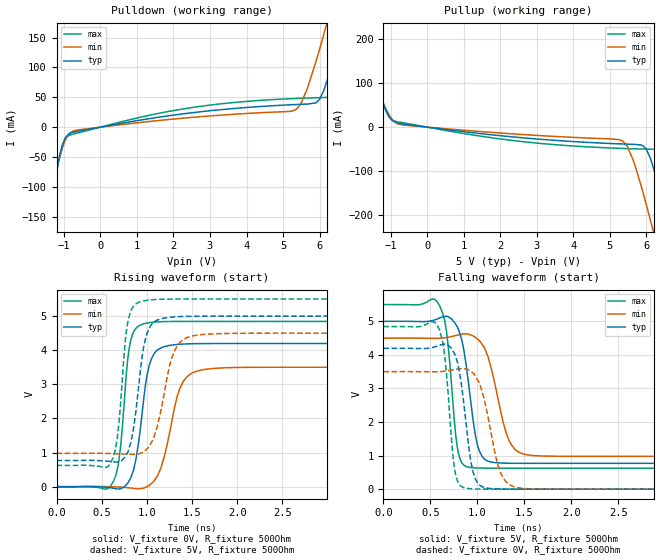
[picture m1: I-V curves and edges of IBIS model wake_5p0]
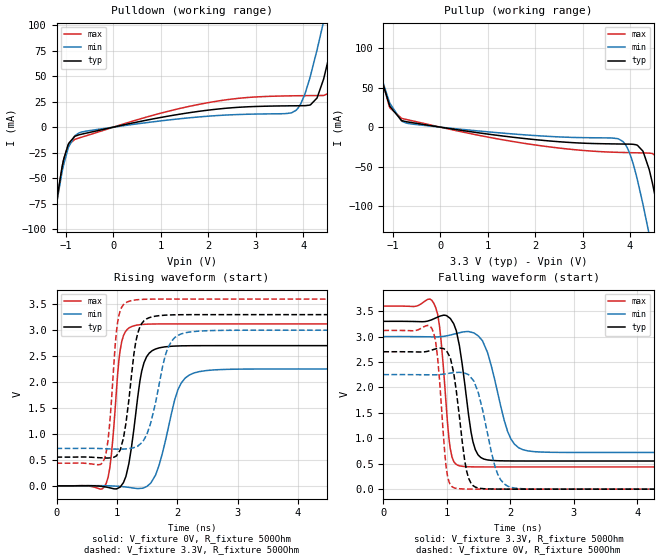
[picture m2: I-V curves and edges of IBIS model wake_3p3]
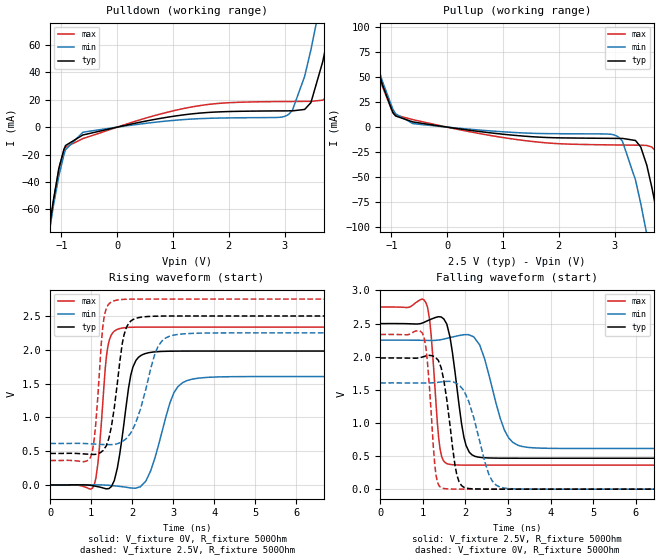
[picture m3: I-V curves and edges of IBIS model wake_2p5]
|Texas Instruments Incorporated
| Marketing part#   Digital Voltage Range   Package-type   #pins
|  TPL5110   1.8V - 5.0V   SOT23   6
[IBIS Ver]   4.1
[File name]   tpl5110.ibs
[File Rev]   1.0
[Date]   09/09/2014
[Source]
| Texas Instruments Incorporated.
| 12500 TI Blvd
| Dallas, TX -75243
[Notes]   Revision History:
| Rev 1.0: 09/09/2014
| - Initial version of the model
| - Model generated from simulations in TISPICE
| - C_comp although listed in numerical order of value are
|   obtained from varying PVT conditions. For PVT conditions for
|   each specific value refer the buffer description under
|   respective [Model]. IBIS model user is responsible for using
|   appropriate C_comp to simulate for Signal Integrity.
| - Warnings regarding combined Non-monotonicity of various models have been
|   reviewd and considered minor and can be ignored.
| - Model names with a trailing _1p8 contains the model for
|   1.8V operation.Model names with a trailing _2p5 contains the model for
|   2.5V operation.Model names with a trailing _3p3 contains the model for
|   3.3V operation.Model names with a trailing _5p0 contains the model
|   for 5.0V operation.
[Disclaimer]
| This model is designed as an aid for customers of Texas Instruments.
| TI and its licensors and suppliers make no warranties, either expressed
| or implied, with respect to this  model, including the warranties of
| merchantability or fitness for a particular purpose. The model is
| provided solely on an "as is" basis. The entire risk as to its quality
| and performance is with the customer.
[Copyright]
 (C) Copyright 2014 Texas Instruments Incorporated.All rights reserved.
|   Device
[Component] TPL5110
[Manufacturer]   TI
[Package]  |
|   typ   min   max
R_pkg   0.067   0.027   0.083
L_pkg   0.937nH   0.593nH   1.143nH
C_pkg   0.144pF   0.126pF   0.200pF
[Pin]  signal_name   model_name   R_pin   L_pin   C_pin
1   VDD   POWER   NA   NA   NA
2   GND   GND   NA   NA   NA
3   EN_oneshot done   NA   NA   NA
4   DONE   done   NA   NA   NA
5   WAKE_MDRV   wake   NA   NA   NA
6   MRST_DELAY   mrst   NA   NA   NA
|   Model Selectors
[Model Selector]  done
done_5p0  done buffer at 5.0V operation
done_3p3  done buffer at 3.3V operation
done_2p5  done buffer at 2.5V operation
done_1p8  done buffer at 1.8V operation
[Model Selector]  mrst
mrst_5p0  mrst buffer at 5.0V operation
mrst_3p3  mrst buffer at 3.3V operation
mrst_2p5  mrst buffer at 2.5V operation
mrst_1p8  mrst buffer at 1.8V operation
[Model Selector]  rstn
rstn_5p0  rstn buffer at 5.0V operation
rstn_3p3  rstn buffer at 3.3V operation
rstn_2p5  rstn buffer at 2.5V operation
rstn_1p8  rstn buffer at 1.8V operation
[Model Selector]  wake
wake_5p0  wake buffer at 5.0V operation
wake_3p3  wake buffer at 3.3V operation
wake_2p5  wake buffer at 2.5V operation
wake_1p8  wake buffer at 1.8V operation
| Models and submodels in the file (16): wake_5p0 (Output), wake_3p3 (Output), wake_2p5 (Output), wake_1p8 (Output), rstn_5p0 (I/O_open_drain), rstn_3p3 (I/O_open_drain), rstn_2p5 (I/O_open_drain), rstn_1p8 (I/O_open_drain), mrst_5p0 (Input), mrst_3p3 (Input), mrst_2p5 (Input), mrst_1p8 (Input), done_5p0 (I/O), done_3p3 (I/O), done_2p5 (I/O), done_1p8 (I/O)
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|   Model
[Model]   wake_5p0
Model_type   Output
Polarity   Non-Inverting
Vmeas = 2.5
Vref = 0
Cref = 1pF
Rref = 100000
|   typ   min   max
C_comp   0.327pF   0.289pF   0.359pF
[Voltage Range]   5   4.5   5.5
[Temperature Range]   25   105   -40
[Pullup Reference]   5   4.5   5.5
[Pulldown Reference]   0   0   0
[Power Clamp Reference]   5   4.5   5.5
[GND Clamp Reference]   0   0   0
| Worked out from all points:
|   slope of the pulldown table from 0 to 0.75 V, typ, clamps not added: 90.8 ohm
|   slope of the pullup table from 0 to 0.75 V, typ, clamps not added: 95.6 ohm
|   falling waveform, V_fixture 5V, R_fixture 500Ohm: 20-80 % time 124ps typ, 177ps min, 91.5ps max; typ from 5 V to 0.769 V
|   rising waveform, V_fixture 0V, R_fixture 500Ohm: 20-80 % time 129ps typ, 183ps min, 95.6ps max; typ from 0 V to 4.2 V
|   rising waveform, V_fixture 5V, R_fixture 500Ohm: 20-80 % time 123ps typ, 173ps min, 92.1ps max; typ from 0.769 V to 5 V
|   falling waveform, V_fixture 0V, R_fixture 500Ohm: 20-80 % time 113ps typ, 160ps min, 84.8ps max; typ from 4.2 V to 0 V
[Pulldown]
|   Voltage   I(typ)   I(min)   I(max)
-5V       -1.486A    -1.386A    -1.583A
-1.595V   -201.3mA   -192.2mA   -216.2mA
-1.43V    -144.2mA   -140.1mA   -154.1mA
-1.025V   -28.11mA   -32.78mA   -28.05mA
-710mV    -8.019mA   -5.887mA   -11.19mA
5.335V    37.79mA    29.02mA    47.98mA
5.905V    41.01mA    110.7mA    49.27mA
6.25V     86.31mA    185.2mA    49.89mA
6.595V    163.7mA    263.5mA    62.44mA
6.955V    251.3mA    347.1mA    139.6mA
7.33V     345.1mA    435.3mA    235.9mA
10V       1.032A     1.077A     962.9mA
[Pullup]
|   Voltage   I(typ)   I(min)   I(max)
-5V       1.028A     955.3mA    1.095A
-2.09V    266.5mA    250.1mA    284mA
-1.655V   156.9mA    149.7mA    165.6mA
-1.085V   30.71mA    34.2mA     29.01mA
-770mV    8.367mA    6.734mA    11.53mA
5.32V     -38.27mA   -30.34mA   -48.45mA
5.905V    -42.54mA   -148.5mA   -49.81mA
6.25V     -108.9mA   -257.7mA   -50.35mA
6.685V    -253.3mA   -403.2mA   -97.13mA
6.955V    -349.7mA   -495.6mA   -188.1mA
7.33V     -486.7mA   -625.3mA   -328.5mA
10V       -1.491A    -1.568A    -1.386A
[Ramp]
R_load = 500
|   typ   min   max
dV/dt_r   2.51801/1.28569e-10   2.10124/1.82749e-10   2.90712/9.55706e-11
dV/dt_f   2.53872/1.23628e-10   2.11358/1.77147e-10   2.92537/9.14795e-11
[Falling Waveform]
V_fixture = 5V
V_fixture_min = 4.5V
V_fixture_max = 5.5V
R_fixture = 500Ohm
C_fixture = 0F
|   Time   V(typ)   V(min)   V(max)
0s        5V         4.5V       5.5V
598ps     5.1V       4.497V     5.469V
672.4ps   5.148V     4.519V     4.695V
785.3ps   4.838V     4.589V     1.276V
913.9ps   2.991V     4.609V     651.2mV
984.6ps   1.53V      4.508V     633.3mV
1.05ns    978.3mV    4.319V     627.8mV
1.336ns   773.4mV    1.464V     624.5mV
1.532ns   769.5mV    1.022V     624.5mV
10ns      768.8mV    977.4mV    624.4mV
[Rising Waveform]
V_fixture = 0V
V_fixture_min = 0V
V_fixture_max = 0V
R_fixture = 500Ohm
C_fixture = 0F
|   Time   V(typ)   V(min)   V(max)
0s        11.88uV    -5.338uV   -17.74uV
632.2ps   -48.36mV   -3.24mV    167.3mV
691.1ps   -65.39mV   -11.2mV    773.4mV
818.4ps   245.1mV    -39.05mV   4.252V
906ps     1.246V     -61.22mV   4.702V
990.3ps   3.07V      -11.5mV    4.792V
1.154ns   4.065V     533.9mV    4.836V
1.403ns   4.182V     3.087V     4.845V
1.659ns   4.195V     3.445V     4.845V
10ns      4.197V     3.502V     4.845V
[Rising Waveform]
V_fixture = 5V
V_fixture_min = 4.5V
V_fixture_max = 5.5V
R_fixture = 500Ohm
C_fixture = 0F
|   Time   V(typ)   V(min)   V(max)
0s        768.8mV    977.4mV    624.4mV
598ps     740.3mV    971.7mV    683.4mV
672.4ps   723.3mV    964.8mV    1.418V
759.4ps   874.6mV    956.6mV    4.228V
800.1ps   1.102V     952.8mV    4.955V
990.3ps   4.391V     1.079V     5.46V
1.116ns   4.884V     1.766V     5.491V
1.308ns   4.978V     3.993V     5.499V
1.532ns   4.997V     4.432V     5.5V
10ns      5V         4.5V       5.5V
[Falling Waveform]
|Gnd
V_fixture = 0V
V_fixture_min = 0V
V_fixture_max = 0V
R_fixture = 500Ohm
C_fixture = 0F
|   Time   V(typ)   V(min)   V(max)
0s        4.197V     3.502V     4.845V
571.1ps   4.261V     3.498V     4.895V
652.5ps   4.32V      3.517V     3.999V
759.4ps   4.021V     3.564V     575.3mV
884.9ps   1.85V      3.576V     24.89mV
947.8ps   590.7mV    3.476V     8.984mV
1.002ns   194.8mV    3.261V     4.297mV
1.253ns   5.124mV    456.9mV    268.3uV
1.44ns    760.1uV    39.68mV    262.3uV
10ns      -8.208uV   6.088uV    -12.22uV
|   Model
[Model]   wake_3p3
Model_type   Output
Polarity   Non-Inverting
Vmeas = 1.65
Vref = 0
Cref = 1pF
Rref = 100000
|   typ   min   max
C_comp   0.327pF   0.289pF   0.359pF
[Voltage Range]   3.3   3   3.6
[Temperature Range]   25   105   -40
[Pullup Reference]   3.3   3   3.6
[Pulldown Reference]   0   0   0
[Power Clamp Reference]   3.3   3   3.6
[GND Clamp Reference]   0   0   0
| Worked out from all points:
|   slope of the pulldown table from 0 to 0.495 V, typ, clamps not added: 100 ohm
|   slope of the pullup table from 0 to 0.495 V, typ, clamps not added: 110 ohm
|   falling waveform, V_fixture 3.3V, R_fixture 500Ohm: 20-80 % time 178ps typ, 274ps min, 123ps max; typ from 3.3 V to 0.554 V
|   rising waveform, V_fixture 0V, R_fixture 500Ohm: 20-80 % time 190ps typ, 285ps min, 131ps max; typ from 0 V to 2.7 V
|   rising waveform, V_fixture 3.3V, R_fixture 500Ohm: 20-80 % time 174ps typ, 261ps min, 122ps max; typ from 0.554 V to 3.3 V
|   falling waveform, V_fixture 0V, R_fixture 500Ohm: 20-80 % time 162ps typ, 243ps min, 113ps max; typ from 2.7 V to 0 V
[Pulldown]
|   Voltage   I(typ)   I(min)   I(max)
-3.3V     -836.9mA   -780.6mA   -895.4mA
-1.33V    -110mA     -109.1mA   -116.7mA
-1.043V   -30.56mA   -35.51mA   -30.38mA
-726mV    -7.503mA   -5.643mA   -10.64mA
1.818V    15.6mA     10.06mA    22.46mA
3.759V    20.91mA    14.12mA    30.69mA
4.026V    21.05mA    31.19mA    30.85mA
4.293V    28.59mA    75.81mA    30.96mA
4.432V    47.18mA    103.7mA    31.04mA
4.719V    106mA      165.6mA    48.26mA
4.957V    161.4mA    219.1mA    98.47mA
6.6V      582.3mA    614.1mA    537.7mA
[Pullup]
|   Voltage   I(typ)   I(min)   I(max)
-3.3V     582.2mA    541.1mA    621.5mA
-1.954V   231mA      217.7mA    245mA
-1.449V   105.8mA    103.4mA    109.8mA
-1.063V   26.2mA     30.06mA    24.31mA
-716.1mV  6.855mA    5.102mA    9.671mA
3.759V    -21.26mA   -14.92mA   -31.85mA
4.026V    -21.53mA   -38.69mA   -32.26mA
4.274V    -30.39mA   -97.65mA   -32.57mA
4.402V    -53.12mA   -135mA     -32.78mA
4.67V     -130.2mA   -218.6mA   -51.93mA
4.986V    -237.9mA   -323mA     -148.9mA
6.6V      -837.2mA   -887.3mA   -774.8mA
[Ramp]
R_load = 500
|   typ   min   max
dV/dt_r   1.62128/1.89539e-10   1.35131/2.85331e-10   1.87269/1.30768e-10
dV/dt_f   1.64785/1.77716e-10   1.36722/2.73675e-10   1.89813/1.22818e-10
[Falling Waveform]
V_fixture = 3.3V
V_fixture_min = 3V
V_fixture_max = 3.6V
R_fixture = 500Ohm
C_fixture = 0F
|   Time   V(typ)   V(min)   V(max)
0s        3.3V       3V         3.6V
795.4ps   3.35V      2.994V     3.653V
883.3ps   3.398V     2.996V     3.218V
1.054ns   3.357V     3.03V      797.3mV
1.207ns   2.752V     3.079V     456.5mV
1.412ns   930.1mV    3.077V     438.6mV
1.636ns   576mV      2.702V     436.7mV
1.958ns   555.5mV    1.135V     436.7mV
2.275ns   553.8mV    752.8mV    436.6mV
10ns      553.6mV    721.3mV    436.4mV
[Rising Waveform]
V_fixture = 0V
V_fixture_min = 0V
V_fixture_max = 0V
R_fixture = 500Ohm
C_fixture = 0F
|   Time   V(typ)   V(min)   V(max)
0s        13.31uV    -8.043uV   8.282uV
823.4ps   -24.22mV   1.276mV    50.33mV
908.5ps   -45.45mV   -1.675mV   594.3mV
1.08ns    16.76mV    -14.35mV   2.78V
1.199ns   429.3mV    -29.93mV   3.041V
1.318ns   1.447V     -49.38mV   3.096V
1.534ns   2.556V     25.13mV    3.118V
2.01ns    2.696V     1.849V     3.121V
2.366ns   2.702V     2.202V     3.121V
10ns      2.702V     2.252V     3.121V
[Rising Waveform]
V_fixture = 3.3V
V_fixture_min = 3V
V_fixture_max = 3.6V
R_fixture = 500Ohm
C_fixture = 0F
|   Time   V(typ)   V(min)   V(max)
0s        553.6mV    721.3mV    436.5mV
795.4ps   536.7mV    715.5mV    523mV
883.3ps   538.2mV    711.7mV    1.232V
1.011ns   609.2mV    707.5mV    3.139V
1.207ns   1.742V     718.6mV    3.559V
1.312ns   2.77V      749.9mV    3.584V
1.412ns   3.129V     830.8mV    3.594V
1.844ns   3.292V     2.654V     3.6V
2.13ns    3.299V     2.949V     3.6V
10ns      3.3V       3V         3.6V
[Falling Waveform]
|Gnd
V_fixture = 0V
V_fixture_min = 0V
V_fixture_max = 0V
R_fixture = 500Ohm
C_fixture = 0F
|   Time   V(typ)   V(min)   V(max)
0s        2.702V     2.252V     3.121V
762.7ps   2.735V     2.249V     3.162V
854.4ps   2.768V     2.251V     2.582V
990.2ps   2.729V     2.269V     420.4mV
1.137ns   2.033V     2.295V     17.97mV
1.281ns   563.6mV    2.283V     3.441mV
1.381ns   114.3mV    2.192V     1.245mV
1.802ns   1.601mV    291.8mV    296uV
2.01ns    366.6uV    36.14mV    288.4uV
10ns      8.873uV    -4.794uV   -5.311uV
|   Model
[Model]   wake_2p5
Model_type   Output
Polarity   Non-Inverting
Vmeas = 1.25
Vref = 0
Cref = 1pF
Rref = 100000
|   typ   min   max
C_comp   0.327pF   0.289pF   0.359pF
[Voltage Range]   2.5   2.25   2.75
[Temperature Range]   25   105   -40
[Pullup Reference]   2.5   2.25   2.75
[Pulldown Reference]   0   0   0
[Power Clamp Reference]   2.5   2.25   2.75
[GND Clamp Reference]   0   0   0
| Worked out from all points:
|   slope of the pulldown table from 0 to 0.375 V, typ, clamps not added: 113 ohm
|   slope of the pullup table from 0 to 0.375 V, typ, clamps not added: 129 ohm
|   falling waveform, V_fixture 2.5V, R_fixture 500Ohm: 20-80 % time 253ps typ, 419ps min, 161ps max; typ from 2.5 V to 0.467 V
|   rising waveform, V_fixture 0V, R_fixture 500Ohm: 20-80 % time 275ps typ, 453ps min, 179ps max; typ from 0 V to 1.98 V
|   rising waveform, V_fixture 2.5V, R_fixture 500Ohm: 20-80 % time 263ps typ, 447ps min, 172ps max; typ from 0.467 V to 2.5 V
|   falling waveform, V_fixture 0V, R_fixture 500Ohm: 20-80 % time 240ps typ, 403ps min, 153ps max; typ from 1.98 V to 0 V
[Pulldown]
|   Voltage   I(typ)   I(min)   I(max)
-2.5V     -533mA     -498.6mA   -571.8mA
-1.195V   -67.5mA    -70.52mA   -70.04mA
-955mV    -16.23mA   -20.15mA   -16.81mA
-617.5mV  -5.736mA   -3.784mA   -8.372mA
1.355V    9.75mA     5.941mA    14.87mA
2.99V     11.87mA    7.726mA    18.68mA
3.14V     11.9mA     12.51mA    18.73mA
3.47V     17.88mA    56.41mA    18.8mA
3.68V     47.48mA    98.82mA    19.66mA
3.882V    89.74mA    143.5mA    39.39mA
4.145V    152.5mA    203.8mA    96.92mA
5V        372.5mA    407.7mA    327.1mA
[Pullup]
|   Voltage   I(typ)   I(min)   I(max)
-2.5V     372.6mA    347.5mA    397.3mA
-1.623V   147mA      141.3mA    154mA
-925mV    11.12mA    13.27mA    12.07mA
57.5mV    -463.9uA   -308.7uA   -674.2uA
2.982V    -11.19mA   -7.658mA   -17.74mA
3.14V     -11.26mA   -14.3mA    -17.84mA
3.373V    -13.3mA    -52.55mA   -17.98mA
3.575V    -37.88mA   -106.6mA   -18.25mA
3.717V    -74.55mA   -149.8mA   -23.05mA
3.845V    -113.6mA   -190.4mA   -44.57mA
4.018V    -171.2mA   -247.1mA   -95.68mA
5V        -533.1mA   -586.2mA   -471.1mA
[Ramp]
R_load = 500
|   typ   min   max
dV/dt_r   1.18847/2.74832e-10   0.962378/4.53253e-10   1.4015/1.79357e-10
dV/dt_f   1.21976/2.52749e-10   0.98154/4.19002e-10   1.43247/1.61207e-10
[Falling Waveform]
V_fixture = 2.5V
V_fixture_min = 2.25V
V_fixture_max = 2.75V
R_fixture = 500Ohm
C_fixture = 0F
|   Time   V(typ)   V(min)   V(max)
0s        2.5V       2.25V      2.75V
1.073ns   2.532V     2.246V     2.814V
1.196ns   2.567V     2.245V     2.314V
1.402ns   2.602V     2.254V     611.7mV
1.564ns   2.487V     2.278V     385.5mV
1.963ns   785mV      2.333V     363.4mV
2.22ns    496.7mV    2.279V     362.9mV
2.916ns   467.5mV    889.9mV    362.8mV
3.229ns   467.1mV    663.7mV    362.8mV
10ns      467.1mV    614.1mV    362.5mV
[Rising Waveform]
V_fixture = 0V
V_fixture_min = 0V
V_fixture_max = 0V
R_fixture = 500Ohm
C_fixture = 0F
|   Time   V(typ)   V(min)   V(max)
0s        1.155uV    906.6nV    -17.53uV
1.073ns   -14.43mV   2.316mV    5.654mV
1.196ns   -29.47mV   1.622mV    537.3mV
1.371ns   -56.36mV   -2.378mV   1.913V
1.618ns   207mV      -15.64mV   2.297V
1.963ns   1.625V     -44.07mV   2.333V
2.295ns   1.94V      35.93mV    2.336V
3.014ns   1.979V     1.365V     2.336V
3.334ns   1.981V     1.544V     2.336V
10ns      1.981V     1.604V     2.336V
[Rising Waveform]
V_fixture = 2.5V
V_fixture_min = 2.25V
V_fixture_max = 2.75V
R_fixture = 500Ohm
C_fixture = 0F
|   Time   V(typ)   V(min)   V(max)
0s        467.1mV    614.1mV    362.5mV
984.5ps   453.1mV    608.7mV    411.6mV
1.111ns   454.8mV    604.4mV    918.6mV
1.308ns   527.2mV    598.2mV    2.461V
1.52ns    981.2mV    598.3mV    2.717V
1.799ns   2.221V     661.6mV    2.746V
2.089ns   2.465V     930mV      2.75V
2.553ns   2.497V     1.945V     2.75V
2.916ns   2.5V       2.202V     2.75V
10ns      2.5V       2.25V      2.75V
[Falling Waveform]
|Gnd
V_fixture = 0V
V_fixture_min = 0V
V_fixture_max = 0V
R_fixture = 500Ohm
C_fixture = 0F
|   Time   V(typ)   V(min)   V(max)
0s        1.981V     1.604V     2.336V
1.028ns   2.003V     1.603V     2.294V
1.111ns   2.017V     1.603V     1.893V
1.279ns   1.997V     1.608V     369.2mV
1.441ns   1.799V     1.62V      19.01mV
1.799ns   213.3mV    1.593V     786.6uV
2.015ns   16.73mV    1.414V     157.3uV
2.553ns   619.2uV    214.7mV    1.709uV
2.818ns   248.7uV    29.41mV    1.063uV
10ns      113.8nV    -897.7nV   -16.46uV
